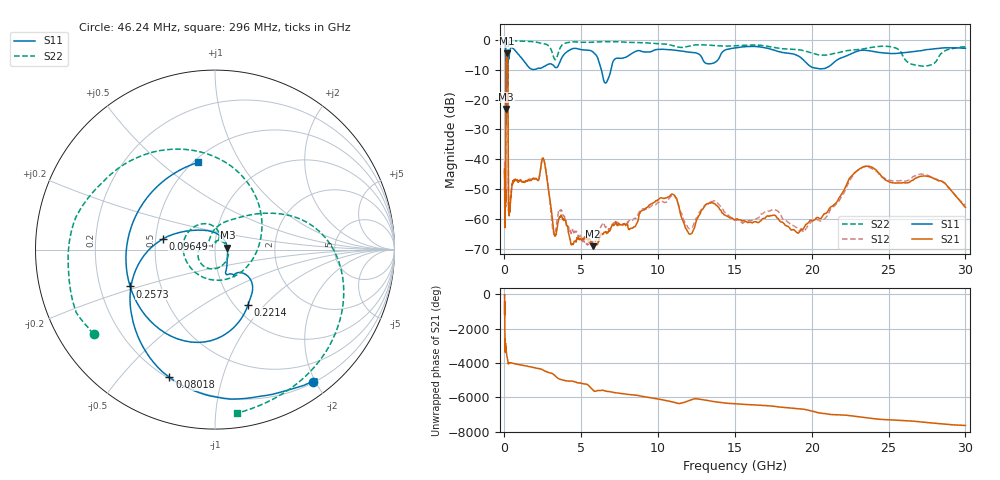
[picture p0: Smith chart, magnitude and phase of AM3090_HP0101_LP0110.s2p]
! Date/Time: Thu, Feb 28, 2019 1:58 PM
! Network Analyzer: Agilent Technologies E8364B Rev: A.07.50.67
! Sweep from 0.010 to 30.000 GHz, 1601 Points, Sweep Type: LOG
! Power Supply: 5.023 V, 0.002 A
# Hz S DB R 50
!freq MagS11 AngS11 MagS21 AngS21 MagS12 AngS12 MagS22 AngS22
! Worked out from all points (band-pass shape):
!   1601 points, 10 MHz to 30 GHz, reference 50 ohm
!   highest |S21| = -4.44 dB at 153.7 MHz (marker M1); lowest = -69.2 dB at 5.783 GHz (marker M2)
!   |S21| within 3 dB of the highest: 107.5 MHz to 211.2 MHz (103.6 MHz wide, 65 % of centre)
!   lowest |S11| = -23.1 dB at 105.1 MHz (marker M3), VSWR 1.15, Z = 57.4 + j1.22 ohm
!   |S11| at or under -10 dB: 96.1 MHz to 213.6 MHz (117.5 MHz wide, 75.9 % of centre); 6.308 GHz to 6.932 GHz (624 MHz wide, 9.43 % of centre)
!   |S22| runs from -28.3 to -0.2 dB; largest |S21 - S12| = 0.014
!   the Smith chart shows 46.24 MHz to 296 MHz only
!   S11 on the Smith chart (normalised r, x): 46.24 MHz: 0.21, -1.97; 80.18 MHz: 0.21, -0.68; 96.49 MHz: 0.55, +0.07; 221.4 MHz: 1.15, -0.81; 257.3 MHz: 0.33, -0.19; 296 MHz: 0.53, +0.68
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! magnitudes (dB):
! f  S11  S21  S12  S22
! 10 MHz  -0.3  -46.1  -40.8  -0.5
! 38.04 MHz  -0.5  -60.1  -60.1  -1.4
! 46.24 MHz  -0.8  -51.4  -51.3  -1.7
! 80.18 MHz  -2.4  -52.2  -52.0  -4.8
! 96.49 MHz  -10.6  -16.6  -16.7  -15.4
! 105.1 MHz  -23.1  -8.4  -8.4  -15.0
! 144.7 MHz  -16.1  -4.5  -4.5  -23.9
! 153.7 MHz  -15.7  -4.4  -4.4  -21.6
! 196.4 MHz  -14.0  -5.6  -5.6  -24.8
! 221.4 MHz  -8.9  -10.6  -10.6  -12.4
! 257.3 MHz  -5.8  -52.3  -50.9  -1.7
! 296 MHz  -6.1  -58.0  -56.9  -0.7
! 550.5 MHz  -2.8  -47.6  -47.6  -0.3
! 2.084 GHz  -9.8  -46.7  -46.5  -0.7
! 2.533 GHz  -9.0  -39.8  -39.7  -1.3
! 3.22 GHz  -8.7  -64.9  -65.2  -6.0
! 5.783 GHz  -4.1  -69.2  -67.5  -0.7
! 7.926 GHz  -5.7  -62.0  -60.9  -0.8
! 10.76 GHz  -3.3  -52.4  -53.0  -1.6
! 19.03 GHz  -5.1  -64.6  -63.0  -3.3
! 23.48 GHz  -3.5  -42.4  -42.5  -2.9
! 30 GHz  -2.8  -56.2  -55.5  -2.3
